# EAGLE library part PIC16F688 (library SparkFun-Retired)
PIC 16F68 8-Bit PIC16F88 RETIRED: IC-07818
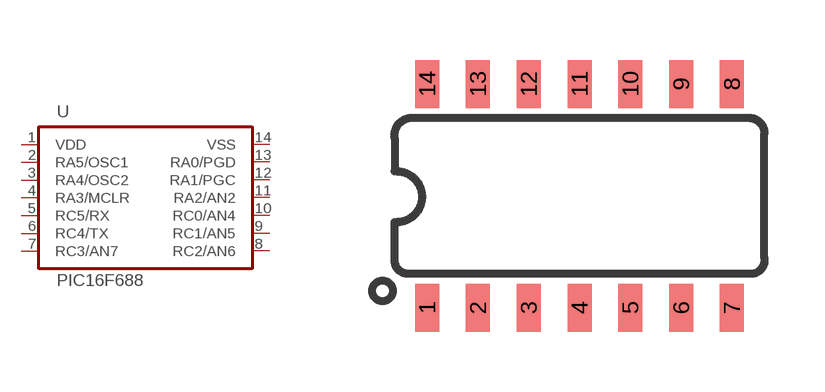
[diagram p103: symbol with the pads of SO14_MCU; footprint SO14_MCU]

Designator prefix -

## PIC16F688SMD  [SO14_MCU]
1  VDD  pwr
2  RA5/OSC1
3  RA4/OSC2
4  RA3/MCLR
5  RC5/RX
6  RC4/TX
7  RC3/AN7
8  RC2/AN6
9  RC1/AN5
10  RC0/AN4
11  RA2/AN2
12  RA1/PGC
13  RA0/PGD
14  VSS  pwr

## Footprint SO14_MCU (pad centres in mm)
SOIC, 0.15 inch width
smd 0.6 x 1.2: 1 -3.175,-2.8; 2 -1.905,-2.8; 3 -0.635,-2.8; 4 0.635,-2.8; 5 1.905,-2.8; 6 3.175,-2.8; 7 4.445,-2.8; 8 4.445,2.8; 9 3.175,2.8; 10 1.905,2.8; 11 0.635,2.8; 12 -0.635,2.8; 13 -1.905,2.8; 14 -3.175,2.8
